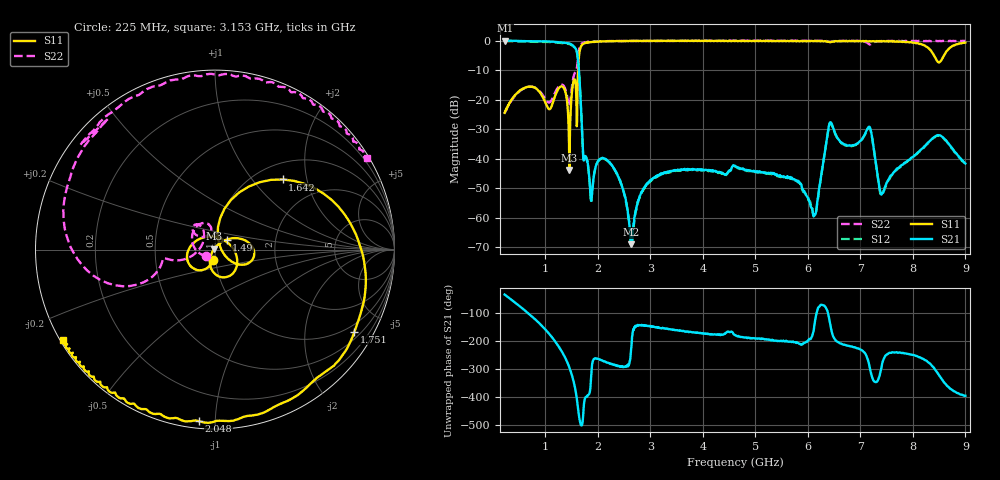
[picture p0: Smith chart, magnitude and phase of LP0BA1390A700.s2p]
!Agilent Technologies,E8358A,US41080443,A.07.50.56
!Agilent E8358A: A.07.50.56
!Date: Monday, May 09, 2016 11:47:23
!Correction: S11(Full 2 Port(1,2))
!S21(Full 2 Port(1,2))
!S12(Full 2 Port(1,2))
!S22(Full 2 Port(1,2))
!S2P File: Measurements: S11, S21, S12, S22:Log Frequency Sweep
# Hz S  dB  R 50
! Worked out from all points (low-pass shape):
!   1601 points, 225 MHz to 9 GHz, reference 50 ohm
!   highest |S21| = -0.01 dB at 227.6 MHz (marker M1); lowest = -69.1 dB at 2.628 GHz (marker M2)
!   |S21| within 3 dB of the highest: start of sweep to 1.585 GHz
!   lowest |S11| = -43.9 dB at 1.46 GHz (marker M3), VSWR 1.01, Z = 49.6 + j0.519 ohm
!   |S11| at or under -10 dB: start of sweep to 1.625 GHz
!   |S22| runs from -24.7 to 0.0 dB; largest |S21 - S12| = 0.021
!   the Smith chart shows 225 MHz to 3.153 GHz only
!   S11 on the Smith chart (normalised r, x): 225 MHz: 0.97, -0.11; 1.49 GHz: 1.13, +0.13; 1.642 GHz: 1.30, +1.44; 1.751 GHz: 0.73, -3.53; 2.048 GHz: 0.04, -0.91; 3.153 GHz: 0.01, -0.28
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2.25e8  -24.52 -99.8  -0.01 -32.4  -0.18 -32.2  -24.66 -144.6
2.276088e8  -24.40 -99.8  -0.01 -32.7  -0.18 -32.5  -24.52 -145.1
6.836016e8  -15.64 -148.7  -0.24 -100.8  -0.41 -100.6  -15.67 128.6
1.074127e9  -23.27 74.1  -0.33 -173.2  -0.50 -173.0  -21.00 120.8
1.340229e9  -15.81 -72.5  -0.75 115.2  -0.91 115.4  -15.14 126.0
1.459576e9  -43.90 125.0  -1.04 65.7  -1.22 65.8  -22.17 162.4
1.490178e9  -21.40 40.8  -1.27 48.6  -1.44 48.8  -18.16 -166.4
1.641694e9  -5.31 46.0  -10.49 -107.5  -10.67 -107.6  -3.19 -167.9
1.687749e9  -1.80 0.4  -25.57 -141.3  -25.69 -141.3  -1.12 163.5
1.75117e9  -0.90 -30.5  -39.54 -46.7  -39.70 -46.9  -0.65 140.3
1.87658e9  -0.57 -69.7  -54.25 44.1  -54.32 45.1  -0.36 128.2
2.048406e9  -0.35 -95.3  -40.03 93.5  -40.15 94.5  -0.25 106.0
2.627574e9  -0.15 -133.3  -69.10 116.8  -67.94 113.3  -0.16 59.0
3.152512e9  -0.13 -149.2  -45.57 -149.8  -45.78 -150.7  -0.10 31.0
4.622431e9  -0.14 -175.2  -42.60 -179.0  -42.79 -178.2  -0.10 -12.5
6.081681e9  -0.17 156.4  -56.83 178.8  -56.69 -177.4  -0.11 -33.1
6.472296e9  -0.33 151.6  -29.13 -177.5  -29.31 -176.5  -0.30 -37.2
7.553438e9  -0.29 134.8  -46.47 119.2  -46.96 116.9  -0.17 -56.0
8.169368e9  -1.30 102.0  -36.71 99.1  -36.91 99.7  -0.17 -68.9
8.417927e9  -5.56 32.0  -32.56 60.5  -32.78 61.0  -0.23 -74.4
8.654074e9  -3.42 -125.0  -34.39 -0.1  -34.47 -0.3  -0.16 -79.8
9e9  -0.71 -176.1  -41.68 -35.0  -41.87 -36.5  -0.18 -85.5
